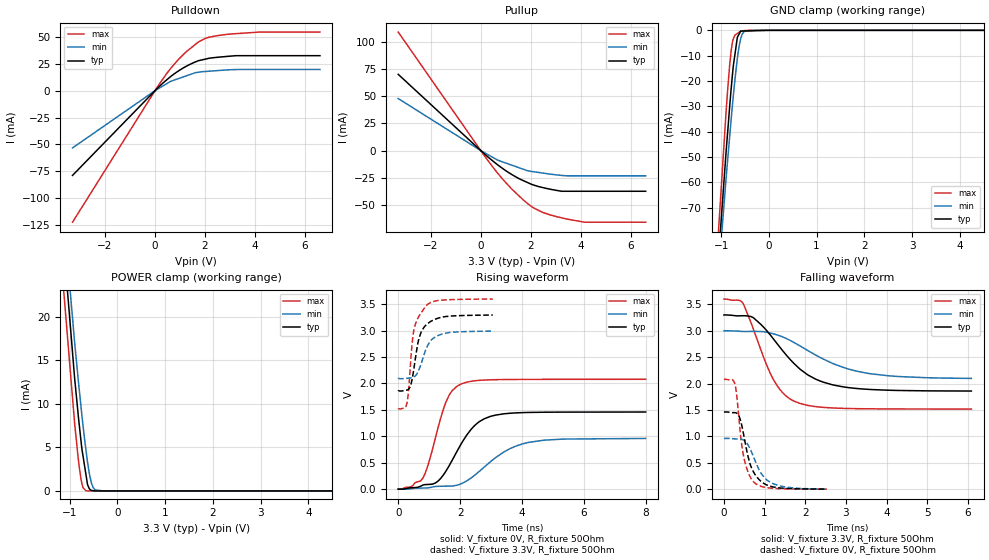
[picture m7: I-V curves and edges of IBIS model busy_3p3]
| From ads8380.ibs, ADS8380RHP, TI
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|   busy_3p3 Model
[Model]   busy_3p3
Model_type   3-state
Polarity   Non-Inverting
Vmeas = 1.65
Vref = 1.65
Cref = 10pF
Rref = 50
|   typ   min   max
|   (nom PVT)   (fast PVT)   (slow PVT)
|C_comp from frequency sweep method (F=1MHz)
|C_comp   3.458e-12   3.339e-12   3.651e-12
|ON state : BUFFER OUTPUT TURNED HIGH
|C_comp   3.458e-12   3.339e-12   3.651e-12
|OFF state: BUFFER IN HIGH IMPEDANCE
|C_comp   2.977e-12   2.823e-12   3.114e-12
|C_comp from LC tank measurement(L=1nH)
C_comp   6.950e-13   6.575e-13   7.409e-13
|Resonant Frequency(Hz)   5.970e+09   6.100e+09   5.800e+09
|C_comp   7.114e-13   6.814e-13   7.537e-13
|ON state : BUFFER OUTPUT TURNED HIGH
|Resonant Frequency(Hz)   5.970e+09   6.100e+09   5.800e+09
|C_comp   7.114e-13   6.814e-13   7.537e-13
|OFF state: BUFFER IN HIGH IMPEDANCE
|Resonant Frequency(Hz)   6.040e+09   6.210e+09   5.850e+09
|C_comp   6.950e-13   6.575e-13   7.409e-13
[Voltage Range]   3.3   3   3.6
[Temperature Range]   35   95   -40
[Pullup Reference]   3.3   3   3.6
[Pulldown Reference]   0   0   0
[Power Clamp Reference]   3.3   3   3.6
[GND Clamp Reference]   0   0   0
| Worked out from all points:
|   slope of the pulldown table from 0 to 0.495 V, typ, clamps not added: 46.6 ohm
|   slope of the pullup table from 0 to 0.495 V, typ, clamps not added: 50.7 ohm
|   GND clamp passes 1 mA (typ) near -0.61 V on its own axis
|   POWER clamp passes 1 mA (typ) near -0.63 V on its own axis
|   falling waveform, V_fixture 3.3V, R_fixture 50Ohm: 20-80 % time 1.06ns typ, 1.43ns min, 683ps max; typ from 3.3 V to 1.86 V
|   rising waveform, V_fixture 0V, R_fixture 50Ohm: 20-80 % time 924ps typ, 1.31ns min, 613ps max; typ from 0 V to 1.46 V
|   rising waveform, V_fixture 3.3V, R_fixture 50Ohm: 20-80 % time 302ps typ, 376ps min, 251ps max; typ from 1.86 V to 3.3 V
|   falling waveform, V_fixture 0V, R_fixture 50Ohm: 20-80 % time 303ps typ, 387ps min, 224ps max; typ from 1.46 V to 0.004 V
[Pulldown]
|   Voltage   I(typ)   I(min)   I(max)
-3.3V     -78.98mA   -53.36mA   -122.6mA
176.4mV   4.073mA    2.487mA    6.361mA
633mV     13.32mA    8.781mA    20.94mA
939.6mV   18.45mA    11.28mA    29.19mA
1.246V    22.71mA    13.78mA    36.21mA
1.706V    27.67mA    17.1mA     44.83mA
2.153V    30.2mA     18.15mA    49.79mA
2.934V    32.05mA    19.43mA    52.68mA
4.162V    32.65mA    19.81mA    54.64mA
6.6V      32.65mA    19.81mA    54.64mA
[GND Clamp]
|   Voltage   I(typ)   I(min)   I(max)
-3.3V     -761.3mA   -676.6mA   -965.4mA
-1.115V   -105.4mA   -111.1mA   -97.09mA
-897.6mV  -48.4mA    -58.78mA   -32.56mA
-856.8mV  -38.65mA   -49.79mA   -21.97mA
-792mV    -23.53mA   -35.54mA   -8.421mA
-766.8mV  -18.32mA   -30.35mA   -5.108mA
-738mV    -13.14mA   -24.6mA    -2.94mA
-660mV    -2.733mA   -11.06mA   -1.235mA
-586.8mV  -322.6uA   -3.017mA   -267.8uA
-510mV    -258uA     -378.2uA   -130.5uA
-285mV    -143.4uA   -450.4nA   -1.904uA
6.6V      0A         0A         0A
[Pullup]
|   Voltage   I(typ)   I(min)   I(max)
-3.3V     69.99mA    47.77mA    108.8mA
18mV      -371.7uA   -256.6uA   -591.9uA
478.8mV   -9.46mA    -6.234mA   -15.01mA
708mV     -13.64mA   -9.093mA   -21.59mA
1.246V    -22.07mA   -13.46mA   -35.43mA
1.89V     -29.57mA   -18.59mA   -48.96mA
2.167V    -32.08mA   -19.64mA   -53.36mA
2.473V    -33.96mA   -20.65mA   -56.75mA
2.812V    -35.67mA   -21.75mA   -59.36mA
3.241V    -37.41mA   -22.85mA   -61.83mA
4.151V    -37.41mA   -23.24mA   -65.82mA
6.6V      -37.41mA   -23.24mA   -65.82mA
[POWER Clamp]
|   Voltage   I(typ)   I(min)   I(max)
-3.3V     298.8mA    244.5mA    432.6mA
-1.156V   30.27mA    33.59mA    24.98mA
-897.6mV  13.01mA    17.12mA    7.827mA
-824.4mV  8.877mA    12.96mA    3.87mA
-766.8mV  5.928mA    9.871mA    1.482mA
-720mV    3.976mA    7.457mA    365.5uA
-662.4mV  1.972mA    4.822mA    28.47uA
-627mV    740.4uA    3.325mA    5.896uA
-549mV    64.5uA     984.1uA    3.448uA
-510mV    36.68uA    395.6uA    2.223uA
-462mV    2.437uA    102.5uA    716.8nA
6.6V      0A         0A         0A
[Ramp]
R_load = 50
|   typ   min   max
dV/dt_r   0.876214/9.23938e-10   0.576036/1.31035e-09   1.24786/6.12367e-10
dV/dt_f   0.864611/1.06042e-09   0.543659/1.44481e-09   1.2486/6.81788e-10
[Falling Waveform]
V_fixture = 3.3V
V_fixture_min = 3V
V_fixture_max = 3.6V
R_fixture = 50Ohm
|   Time   V(typ)   V(min)   V(max)
0s        3.3V       3V         3.6V
466ps     3.286V     2.988V     3.526V
724ps     3.249V     2.99V      3.034V
1.02ns    3.032V     2.979V     2.413V
1.228ns   2.836V     2.94V      2.062V
1.452ns   2.618V     2.882V     1.823V
1.714ns   2.389V     2.784V     1.673V
2.332ns   2.061V     2.51V      1.559V
3.372ns   1.901V     2.219V     1.525V
6.088ns   1.86V      2.099V     1.519V
[Rising Waveform]
V_fixture = 0V
V_fixture_min = 0V
V_fixture_max = 0V
R_fixture = 50Ohm
|   Time   V(typ)   V(min)   V(max)
0s        1.371nV    3.229nV    1.196nV
794ps     76.83mV    21.38mV    206.9mV
970ps     89.68mV    25.69mV    469.8mV
1.24ns    131.7mV    52.31mV    1.056V
1.548ns   347.7mV    56.8mV     1.656V
1.744ns   547.3mV    59.32mV    1.864V
2.042ns   864.5mV    104.2mV    1.992V
2.78ns    1.332V     418.4mV    2.066V
4.08ns    1.45V      866.6mV    2.077V
7.998ns   1.46V      960.1mV    2.08V
[Rising Waveform]
V_fixture = 3.3V
V_fixture_min = 3V
V_fixture_max = 3.6V
R_fixture = 50Ohm
|   Time   V(typ)   V(min)   V(max)
0s        1.858V     2.092V     1.519V
264ps     1.874V     2.097V     1.589V
334ps     1.892V     2.103V     1.868V
438ps     2.049V     2.111V     2.684V
502ps     2.261V     2.12V      2.997V
672ps     2.855V     2.266V     3.276V
886ps     3.099V     2.633V     3.461V
1.072ns   3.182V     2.826V     3.541V
1.41ns    3.254V     2.935V     3.578V
3.056ns   3.296V     2.992V     3.598V
[Falling Waveform]
V_fixture = 0V
V_fixture_min = 0V
V_fixture_max = 0V
R_fixture = 50Ohm
|   Time   V(typ)   V(min)   V(max)
0s        1.461V     961.6mV    2.08V
264ps     1.452V     955.4mV    2.007V
300ps     1.447V     953.3mV    1.868V
368ps     1.393V     951.8mV    1.353V
486ps     1.031V     932.5mV    615.5mV
632ps     506.7mV    785.7mV    255.8mV
722ps     336.2mV    627.5mV    147.4mV
928ps     140.1mV    287.5mV    52.15mV
1.214ns   44.46mV    105.9mV    18.8mV
2.53ns    3.708mV    5.357mV    2.77mV
